(* Logix 5000 DataType export CM1T_CMLDriveStatus; software revision 20.00 *)

TYPE CM1T_CMLDriveStatus :
STRUCT
   StatusValue : SINT;   // Indicates status and error type
   StatusValue1 : SINT;   // Additional status values
   In_Position : BOOL;   // Drive is in position and ready to move
   Moving : BOOL;   // Drive is currently moving
   Disabled : BOOL;   // Drive is disabled
   Error : BOOL;   // Drive is in an error state
   HomeAchieved : BOOL;   // Home achieved
END_STRUCT
END_TYPE
